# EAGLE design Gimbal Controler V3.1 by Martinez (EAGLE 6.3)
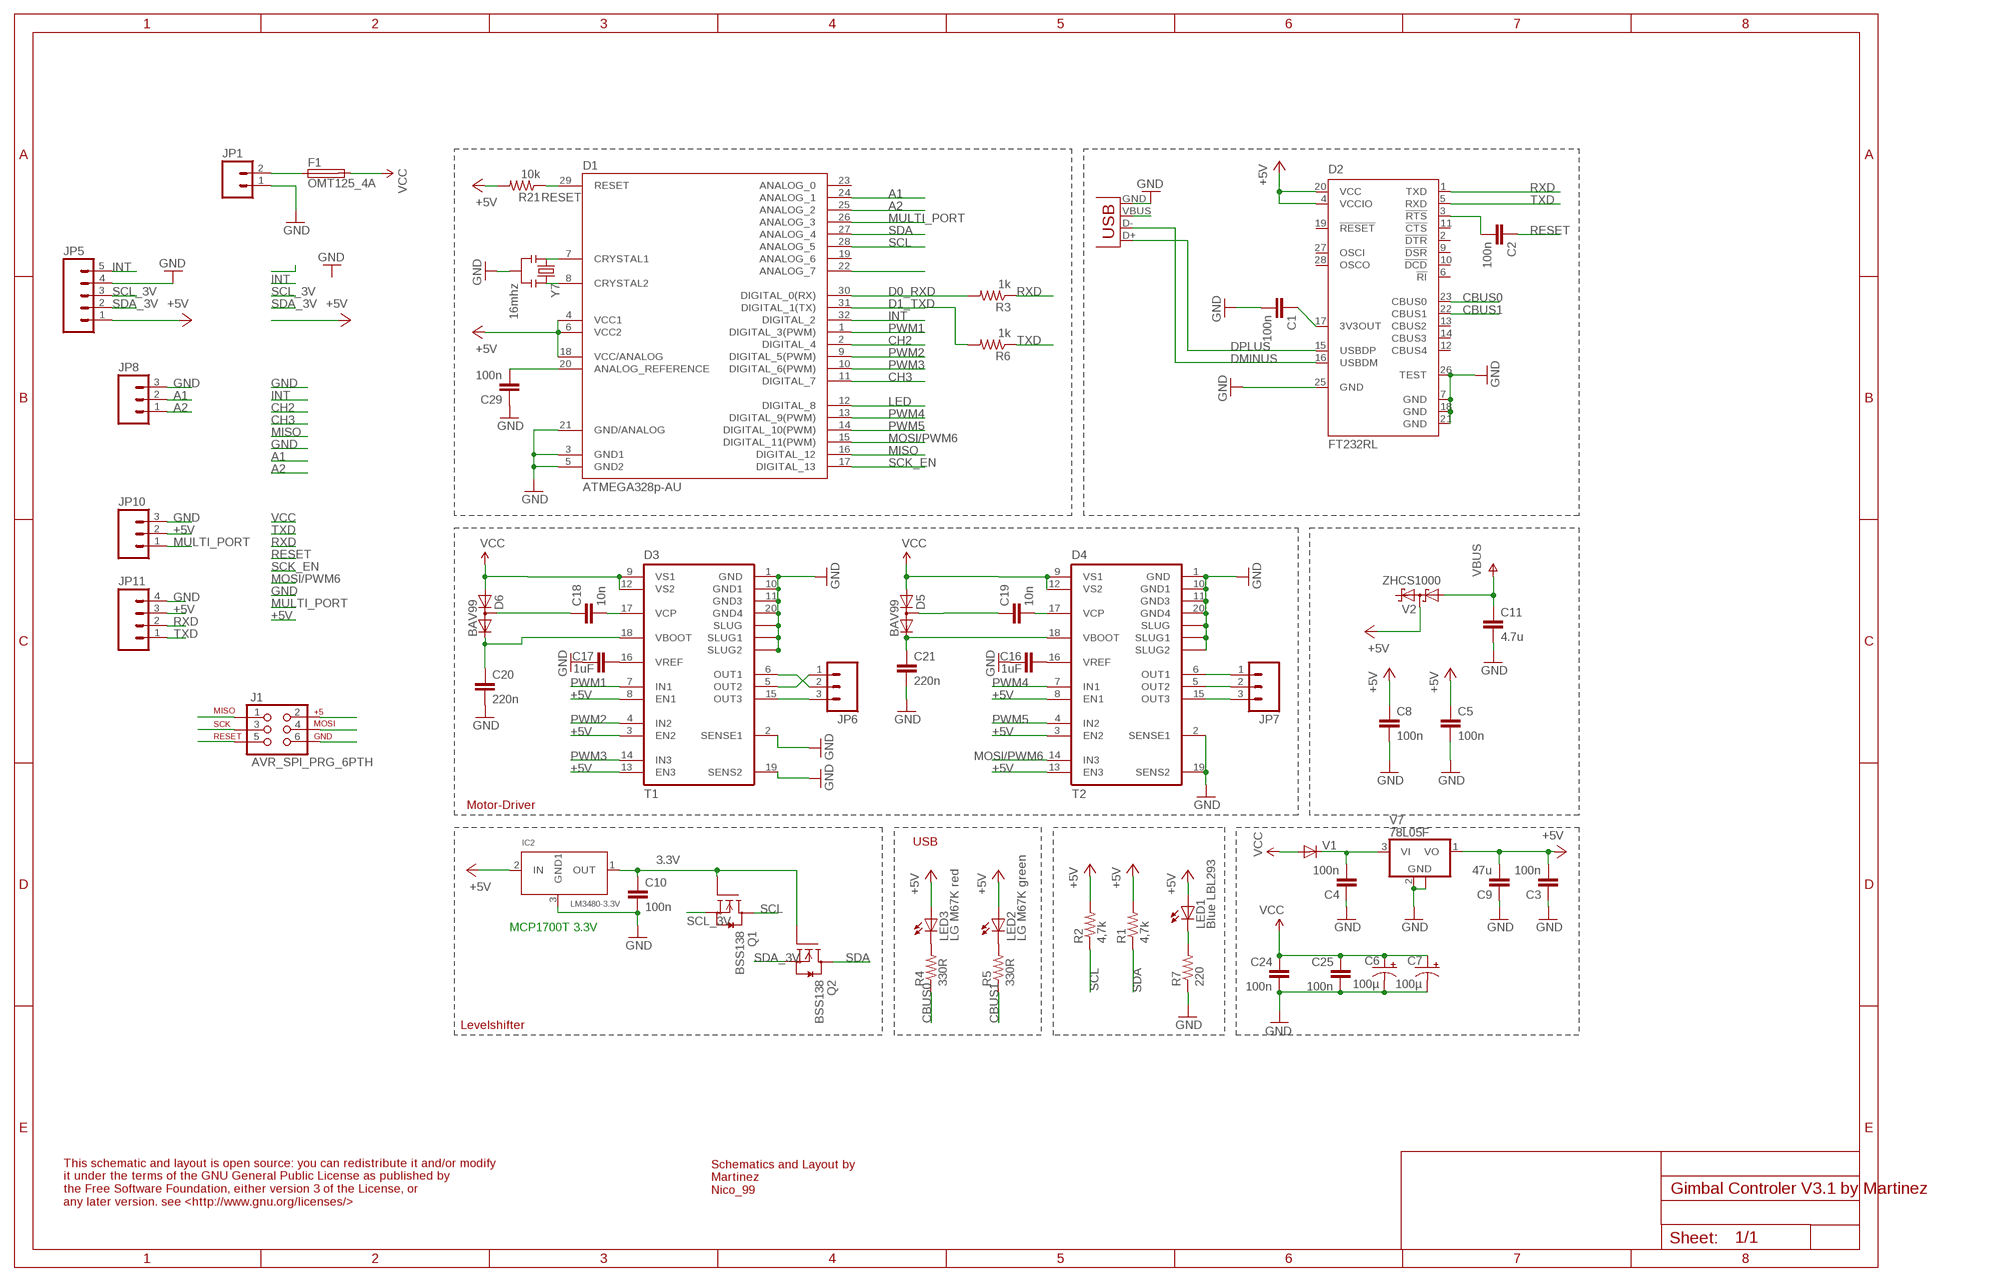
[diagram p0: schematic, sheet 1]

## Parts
C1  100n  CAP0805  [0805]
C2  100n  CAP0805  [0805]
C3  100n  CAP0805  [0805]
C4  100n  CAP0805  [0805]
C5  100n  CAP0805  [0805]
C6  100µ  CAP_POLD  [PANASONIC_D]
C7  100µ  CAP_POLD  [PANASONIC_D]
C8  100n  CAP0805  [0805]
C9  47u  C-EUC1210  [C1210]
C10  100n  CAP0805  [0805]
C11  4.7u  CAP0805  [0805]
C16  1uF  CAP0805  [0805]
C17  1uF  CAP0805  [0805]
C18  10n  CAP0805  [0805]
C19  10n  CAP0805  [0805]
C20  220n  CAP0805  [0805]
C21  220n  CAP0805  [0805]
C24  100n  CAP0805  [0805]
C25  100n  CAP0805  [0805]
C29  100n  CAP0805  [0805]
D1  ATMEGA328p-AU  ATMEGA168-AU  [TQFP32-08]
D2  FT232RL  [SSOP28]
D3  T1  L6234  [SO20POWER2]
D4  T2  L6234  [SO20POWER2]
D5  BAV99  BAV199  [SOT23]
D6  BAV99  BAV199  [SOT23]
F1  OMT125_4A  OMT125_11MM  [OMT125_11MM]
IC2  LM3480-3.3V  VREG_MULTI2  [SOT23]
J1  AVR_SPI_PRG_6PTH  [2X3]
JP1  M02PTH  [1X02]
JP5  M05PTH  [1X05]
JP6  M03PTH  [1X03]
JP7  M03PTH  [1X03]
JP8  M031X03_NO_SILK  [1X03_NO_SILK]
JP10  M031X03_NO_SILK  [1X03_NO_SILK]
JP11  M041X04_NO_SILK  [1X04_NO_SILK]
LED1  Blue LBL293  LEDCHIP-LED0603  [CHIP-LED0603]
LED2  LG M67K green  LEDCHIP-LED0805  [CHIP-LED0805]
LED3  LG M67K red  LEDCHIP-LED0805  [CHIP-LED0805]
Q1  BSS138  [SOT23]
Q2  BSS138  [SOT23]
R1  4,7k  RESISTOR0805-RES  [0805]
R2  4,7k  RESISTOR0805-RES  [0805]
R3  1k  RESISTOR0805-RES  [0805]
R4  330R  RESISTOR0805-RES  [0805]
R5  330R  RESISTOR0805-RES  [0805]
R6  1k  RESISTOR0805-RES  [0805]
R7  220  RESISTOR0805-RES  [0805]
R21  10k  RESISTOR0805-RES  [0805]
V1  DIODE-DO214AC  [DO214AC]
V2  ZHCS1000  BAS40-04  [SOT23]
V7  78L05F  [SOT89]
X2  USBOLD  [USB-MINIB-OLD]
Y7  16mhz  RESONATORSMD  [RESONATOR-SMD]

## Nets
3.3V: C10.1 IC2.1(OUT) Q1.1(G) Q2.1(G)
+5V: C3.2 C5.1 C8.1 C9.2 D1.4(VCC1) D1.6(VCC2) D1.18(VCC/ANALOG) D2.4(VCCIO) D2.20(VCC) D3.3(EN2) D3.8(EN1) D3.13(EN3) D4.3(EN2) D4.8(EN1) D4.13(EN3) IC2.2(IN) J1.2 JP5.1 JP10.2 JP11.3 LED1.A LED2.A LED3.A R1.2 R2.2 R21.2 V2.3(C1A2) V7.1(VO)
A1: D1.24(ANALOG_1) JP8.2
A2: D1.25(ANALOG_2) JP8.1
A7: D1.22(ANALOG_7)
CBUS0: D2.23(CBUS0) R4.1
CBUS1: D2.22(CBUS1) R5.1
CH2: D1.2(DIGITAL_4)
CH3: D1.11(DIGITAL_7)
D0_RXD: D1.30(DIGITAL_0(RX)) R3.2
D1_TXD: D1.31(DIGITAL_1(TX)) R6.2
DMINUS: D2.16(USBDM) X2.D-
DPLUS: D2.15(USBDP) X2.D+
GND: C1.2 C3.1 C4.1 C5.2 C6.- C7.- C8.2 C9.1 C10.2 C11.2 C16.1 C17.1 C20.2 C21.2 C24.2 C25.2 C29.1 D1.3(GND1) D1.5(GND2) D1.21(GND/ANALOG) D2.7(GND) D2.18(GND) D2.21(GND) D2.25(GND) D2.26(TEST) D3.1(GND) D3.2(SENSE1) D3.10(GND1) D3.11(GND3) D3.19(SENS2) D3.20(GND4) D3.SLUG1(SLUG2) D3.SLUG2(SLUG) D3.SLUG(SLUG1) D4.1(GND) D4.2(SENSE1) D4.10(GND1) D4.11(GND3) D4.19(SENS2) D4.20(GND4) D4.SLUG1(SLUG2) D4.SLUG2(SLUG) D4.SLUG(SLUG1) IC2.3(GND1) J1.6 JP1.1 JP5.4 JP8.3 JP10.3 JP11.4 R7.1 V7.2(GND) V7.2@1(GND) X2.GND Y7.2
INT: D1.32(DIGITAL_2) JP5.5
LED: D1.12(DIGITAL_8)
MISO: D1.16(DIGITAL_12) J1.1
MOSI/PWM6: D1.15(DIGITAL_11(PWM)) D4.14(IN3) J1.4
MULTI_PORT: D1.26(ANALOG_3) JP10.1
N$1: LED3.C R4.2
N$2: LED2.C R5.2
N$3: F1.P$1 JP1.2
N$4: LED1.C R7.2
N$7: C16.2 D4.16(VREF)
N$8: C17.2 D3.16(VREF)
N$17: C18.2 D3.17(VCP)
N$18: C19.2 D4.17(VCP)
N$19: C19.1 D5.3(AC)
N$20: C21.1 D4.18(VBOOT) D5.2(C)
N$21: D3.15(OUT3) JP6.3
N$22: C1.1 D2.17(3V3OUT)
N$23: D4.6(OUT1) JP7.1
N$24: D4.5(OUT2) JP7.2
N$25: D4.15(OUT3) JP7.3
N$26: C2.2 D2.3(!RTS)
N$27: D3.5(OUT2) JP6.1
N$28: D3.6(OUT1) JP6.2
N$38: D1.8(CRYSTAL2) Y7.3
N$39: D1.7(CRYSTAL1) Y7.1
N$40: C29.2 D1.20(ANALOG_REFERENCE)
PWM1: D1.1(DIGITAL_3(PWM)) D3.7(IN1)
PWM2: D1.9(DIGITAL_5(PWM)) D3.4(IN2)
PWM3: D1.10(DIGITAL_6(PWM)) D3.14(IN3)
PWM4: D1.13(DIGITAL_9(PWM)) D4.7(IN1)
PWM5: D1.14(DIGITAL_10(PWM)) D4.4(IN2)
RESET: C2.1 D1.29(RESET) J1.5 R21.1
RXD: D2.1(TXD) JP11.2 R3.1
SCK_EN: D1.17(DIGITAL_13) J1.3
SCL: D1.28(ANALOG_5) Q1.3(D) R2.1
SCL_3V: JP5.3 Q1.2(S)
SDA: D1.27(ANALOG_4) Q2.3(D) R1.1
SDA_3V: JP5.2 Q2.2(S)
TXD: D2.5(RXD) JP11.1 R6.1
VBOOT1: C20.1 D3.18(VBOOT) D6.2(C)
VBUS: C11.1 V2.1(A1) X2.VBUS
VCC: C6.+ C7.+ C24.1 C25.1 D3.9(VS1) D3.12(VS2) D4.9(VS1) D4.12(VS2) D5.1(A) D6.1(A) F1.P$2 V1.A
VCC_VI: C4.2 V1.C V7.3(VI)
VCP1: C18.1 D6.3(AC)
Unconnected: D1.19(ANALOG_6) D1.23(ANALOG_0) D2.2(!DTR) D2.6(!RI) D2.9(!DSR) D2.10(!DCD) D2.11(!CTS) D2.12(CBUS4) D2.13(CBUS2) D2.14(CBUS3) D2.19(!RESET) D2.27(OSCI) D2.28(OSCO) V2.2(C2)

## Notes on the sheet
- FTDI
- Motor-Driver
- USB
- MCP1700T 3.3V
- Levelshifter
- Schematics and Layout by
  Martinez
  Nico_99
- This schematic and layout is open source: you can redistribute it and/or modify
  it under the terms of the GNU General Public License as published by
  the Free Software Foundation, either version 3 of the License, or
  any later version. see <http://www.gnu.org/licenses/>

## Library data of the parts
C1-C5 C8 C10 C11 C16-C21 C24 C25 C29 = SparkFun:CAP: Capacitor
C6 C7 = SparkFun:CAP_POL: Capacitor Polarized
C9 = rcl:C-EU: CAPACITOR, European symbol
D1 = Arduino-AVR:ATMEGA168
D2 = ftdichip:FT232R: Source: http://www.ftdichip.com/Documents/DataSheets/DS_FT232R_v104.pdf; MPN: FT232RL; OC_FARNELL: 1146032; OC_NEWARK: 91K9918
D3 D4 = L6234:L6234
D5 D6 = diode:BAV199: DIODE low-leakage double diode
F1 = fuse:OMT125_11MM
IC2 = m-pad-2.1_my:VREG_MULTI2: standard package voltage regulator (LM3480, etc)
J1 = SparkFun:AVR_SPI_PRG_6: AVR ISP 6 Pin This is the reduced ISP connector for AVR programming. Common on Arduino. This footprint will take up less PCB space and can be used with a 10-pin to 6-pin adapter such as SKU: BOB-08508
JP1 = SparkFun:M02: Header 2
JP5 = SparkFun:M05: Header 5 Standard 5-pin 0.1" header. Use with straight break away headers (SKU : PRT-00116), right angle break away headers (PRT-00553), swiss pins (PRT-00743), machine pins (PRT-00117), and female headers (PRT-00115). Molex polarized connector foot print use with SKU : PRT-08230 with associated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
JP6-JP8 JP10 = SparkFun:M03: Header 3 Standard 3-pin 0.1" header. Use with straight break away headers (SKU : PRT-00116), right angle break away headers (PRT-00553), swiss pins (PRT-00743), machine pins (PRT-00117), and female headers (PRT-00115). Molex polarized connector foot print use with SKU : PRT-08232 with associated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
JP11 = SparkFun:M04: Header 4 Standard 4-pin 0.1" header. Use with straight break away headers (SKU : PRT-00116), right angle break away headers (PRT-00553), swiss pins (PRT-00743), machine pins (PRT-00117), and female headers (PRT-00115). Molex polarized connector foot print use with SKU : PRT-08231 with associated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
LED1-LED3 = led:LED: LED
Q1 Q2 = m-pad-2.1_my:BSS138: Fairchild Semiconductors BSS138 N-Channel Logic Level Enhancement Mode Field Effect Transistor General Description: These N-Channel enhancement mode field effect transistors are produced using Fairchild's proprietary, high cell density, DMOS technology. These products have been designed to minimize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
R1-R7 R21 = SparkFun:RESISTOR: Resistor
V1 = diode:DIODE-: DIODE
V2 = diode:BAS40-04: Silicon Schottky Diodes General-purpose diode for high-speed switching
V7 = linear:78L*: POSITOIV-VOLTAGE REGULATORS Output up to 100 mA Source: http://focus.ti.com/lit/ds/symlink/ua78l05.pdf
X2 = SparkFun:USB: USB Connectors USB-B-PTH is fully proven SKU : PRT-00139 USB-miniB is fully proven SKU : PRT-00587 USB-A-PCB is untested. USB-A-H is throughly reviewed, but untested. Spark Fun Electronics SKU : PRT-00437 USB-B-SMT is throughly reviewed, but untested. Needs silkscreen touching up. USB-A-S has not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
Y7 = SparkFun:RESONATOR: Resonator Small SMD resonator. This is the itty bitty 10/20MHz resonators with built in caps. CSTCE10M0G55 and CSTCE20M0V53. Footprint has been reviewed closely but hasn't been tested yet.

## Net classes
0 default: width 0.152 mm, clearance 0.152 mm

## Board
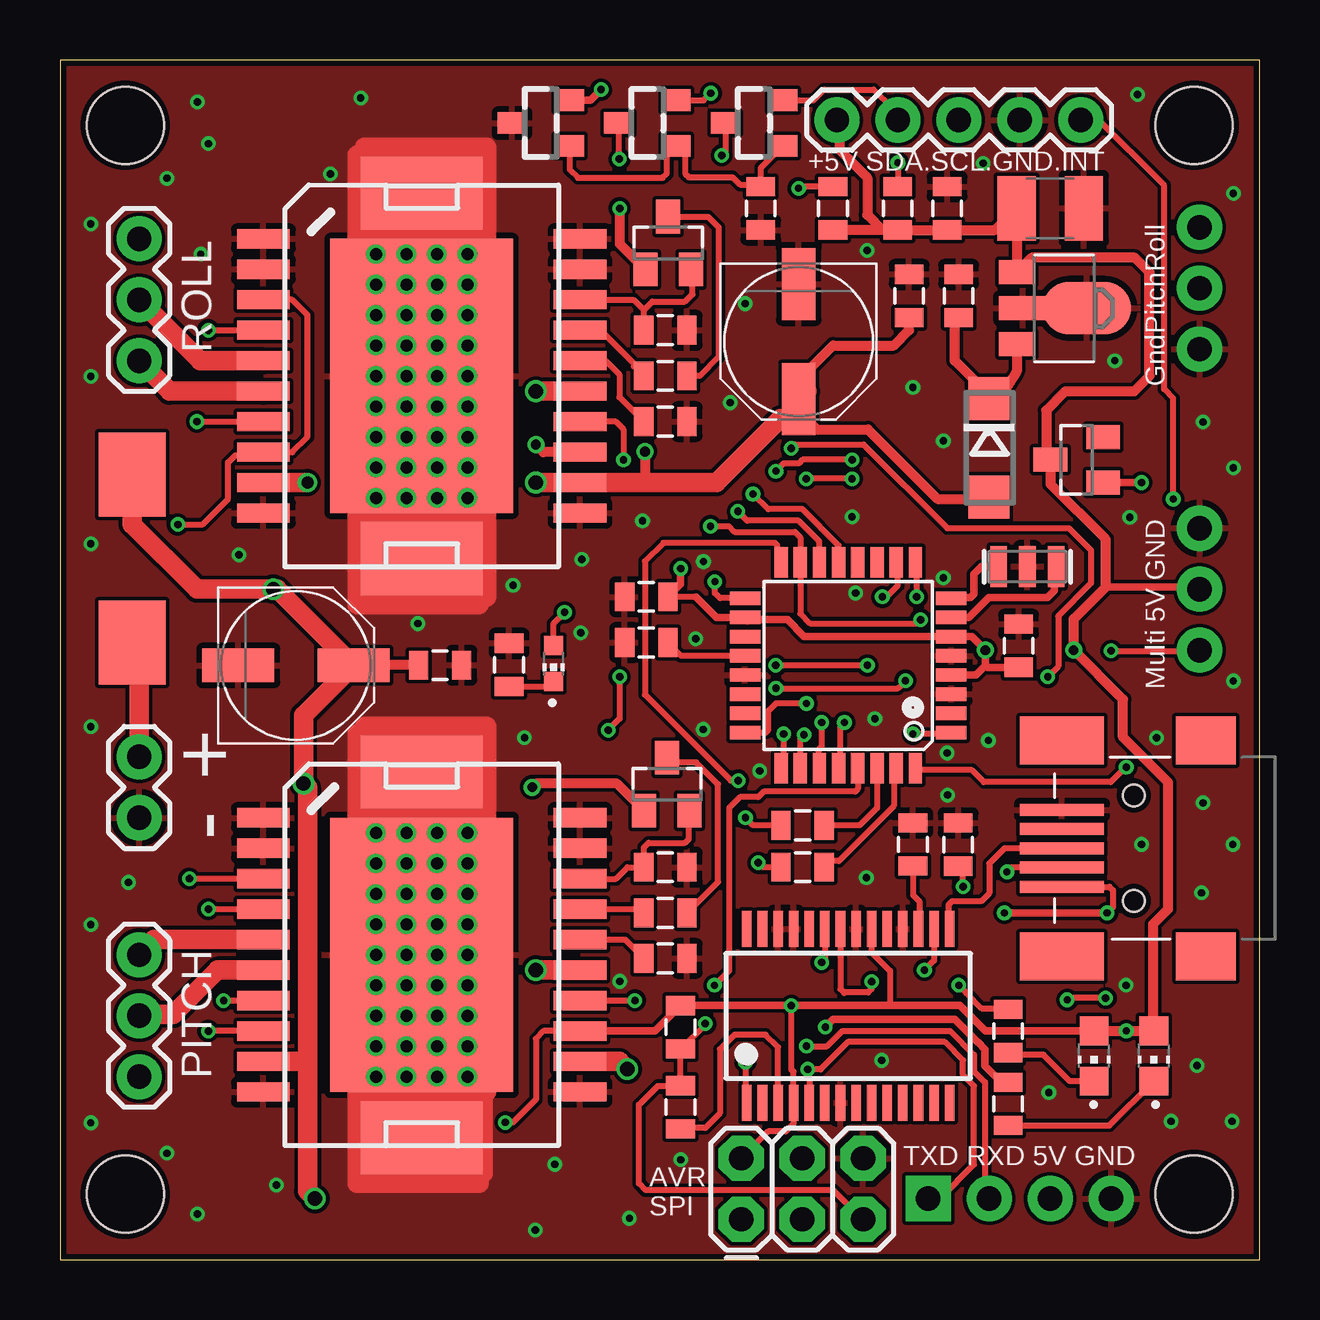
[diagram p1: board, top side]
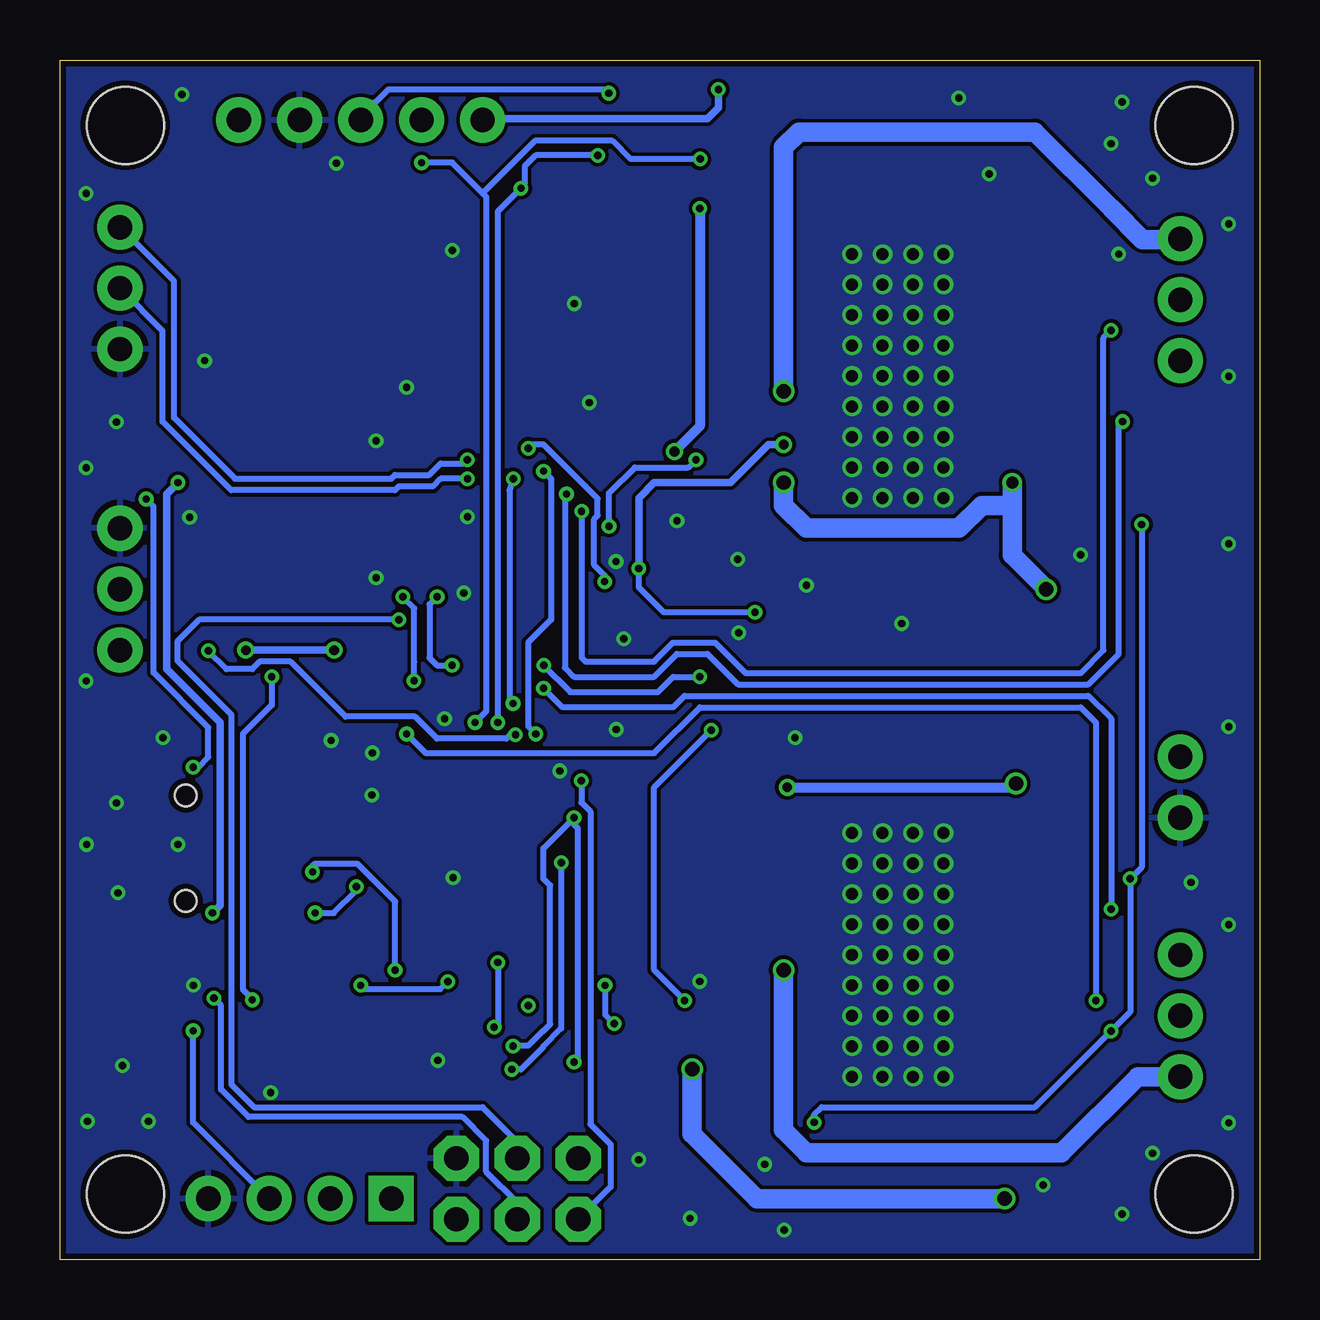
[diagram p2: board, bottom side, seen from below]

Size 50 x 50 mm. Coordinates in mm from the lower left corner, seen from the top.
Outline: 50,0 50,50 0,50 0,0 50,0
Copper layers (1*16): Top 0.035mm / dielectric 1.5mm / Bottom 0.035mm
Design rules "ITEADstudio_DRC *": minimum track width 6mil, minimum drill 12mil, track to track 6mil, track to pad 6mil, pad to pad 6mil, via to via 6mil, smd to smd 0mil, copper to edge 10mil, drill to drill 10mil, minimum pad ring 10mil, minimum via ring 6mil, stop-mask expansion 2mil, vias tented up to drill 100mil, thermal gap 10mil
Holes 3.2 mm at 47.27,2.73 2.73,2.73 2.73,47.27 47.27,47.27

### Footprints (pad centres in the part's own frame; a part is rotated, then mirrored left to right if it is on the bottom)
0805 = smd 0.8 x 1.2: 1 -0.9,0; 2 0.9,0
PANASONIC_D = smd 3 x 1.4: + 2.4,0; - -2.4,0
C1210 = smd 1.6 x 2.7: 1 -1.4,0; 2 1.4,0
TQFP32-08 = smd 1.27 x 0.559: 1 -4.293,2.8; 2 -4.293,2; 3 -4.293,1.2; 4 -4.293,0.4; 5 -4.293,-0.4; 6 -4.293,-1.2; 7 -4.293,-2; 8 -4.293,-2.8; 17 4.293,-2.8; 18 4.293,-2; 19 4.293,-1.2; 20 4.293,-0.4; 21 4.293,0.4; 22 4.293,1.2; 23 4.293,2; 24 4.293,2.8 | smd 0.559 x 1.27: 9 -2.8,-4.293; 10 -2,-4.293; 11 -1.2,-4.293; 12 -0.4,-4.293; 13 0.4,-4.293; 14 1.2,-4.293; 15 2,-4.293; 16 2.8,-4.293; 25 2.8,4.293; 26 2,4.293; 27 1.2,4.293; 28 0.4,4.293; 29 -0.4,4.293; 30 -1.2,4.293; 31 -2,4.293; 32 -2.8,4.293
SSOP28 = smd 0.4 x 1.5: 1 -4.225,-3.625; 2 -3.575,-3.625; 3 -2.925,-3.625; 4 -2.275,-3.625; 5 -1.625,-3.625; 6 -0.975,-3.625; 7 -0.325,-3.625; 8 0.325,-3.625; 9 0.975,-3.625; 10 1.625,-3.625; 11 2.275,-3.625; 12 2.925,-3.625; 13 3.575,-3.625; 14 4.225,-3.625; 15 4.225,3.625; 16 3.575,3.625; 17 2.925,3.625; 18 2.275,3.625; 19 1.625,3.625; 20 0.975,3.625; 21 0.325,3.625; 22 -0.325,3.625; 23 -0.975,3.625; 24 -1.625,3.625; 25 -2.275,3.625; 26 -2.925,3.625; 27 -3.575,3.625; 28 -4.225,3.625
SO20POWER2 = smd 0.8 x 2.2: 1 -5.715,-6.6; 2 -4.445,-6.6; 3 -3.175,-6.6; 4 -1.905,-6.6; 5 -0.635,-6.6; 6 0.635,-6.6; 7 1.905,-6.6; 8 3.175,-6.6; 9 4.445,-6.6; 10 5.715,-6.6; 11 5.715,6.6; 12 4.445,6.6; 13 3.175,6.6; 14 1.905,6.6; 15 0.635,6.6; 16 -0.635,6.6; 17 -1.905,6.6; 18 -3.175,6.6; 19 -4.445,6.6; 20 -5.715,6.6 | smd 3.048 x 5.08: SLUG -7.62,0; SLUG2 7.62,0 | smd 11.43 x 7.62: SLUG1 0,0
SOT23 = smd 1 x 1.4: 1 -0.95,-1.1; 2 0.95,-1.1; 3 0,1.1
OMT125_11MM = smd 3.5 x 2.8: P$1 -3.5,0; P$2 3.5,0
SOT23' = smd 0.9 x 1.2: 1 -0.95,-1.2; 2 0.95,-1.2; 3 0,1.2
2X3 = drill 1.016 pad 1.88 octagon: 1 0,0; 2 0,2.54; 3 2.54,0; 4 2.54,2.54; 5 5.08,0; 6 5.08,2.54
1X02 = drill 1.016 pad 1.88: 1 0,0; 2 2.54,0
1X05 = drill 1.016 pad 1.88: 1 0,0; 2 2.54,0; 3 5.08,0; 4 7.62,0; 5 10.16,0
1X03 = drill 1.016 pad 1.88: 1 0,0; 2 2.54,0; 3 5.08,0
1X03_NO_SILK = drill 1.016 pad 1.88: 1 0,0; 2 2.54,0; 3 5.08,0
1X04_NO_SILK = drill 1.016 pad 1.88 square: 1 0,0 | drill 1.016 pad 1.88: 2 2.54,0; 3 5.08,0; 4 7.62,0
CHIP-LED0603 = smd 0.8 x 0.8: A 0,-0.75; C 0,0.75
CHIP-LED0805 = smd 1.2 x 1.2: A 0,-1.05; C 0,1.05
DO214AC = smd 1.8 x 1.7: A 2.05,0; C -2.05,0
SOT89 = smd 1 x 1.5: 1 -1.499,-1.981; 3 1.499,-1.981 | smd 1 x 2: 2 0,-1.727 | smd 2.2 x 3.7: 2@1 0,0.94
USB-MINIB-OLD = smd 2.5 x 2: 1 -3,-4.5; 2 -3,4.5 | smd 3.5 x 2: 3 3,-4.5; 4 3,4.5 | smd 3.5 x 0.5: D+ 3,0; D- 3,0.8; GND 3,-1.6; ID 3,-0.8; VBUS 3.01,1.61 | hole 0.9: 0,2.2; 0,-2.2
RESONATOR-SMD = smd 0.7 x 1.7: 1 -1.2,0; 2 0,0; 3 1.2,0

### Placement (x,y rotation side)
C1  35.55,17.3 90 top
C2  25.87,6.35 270 top
C3  36.98,43.81 270 top
C4  37.46,40.16 270 top
C5  24.44,27.62 180 top
C6  9.84,24.77 0 top
C7  30.79,38.26 270 top
C8  39.96,25.58 90 top
C9  41.27,43.81 180 top
C10  29.21,43.81 270 top
C11  37.44,17.3 90 top
C16  25.23,34.92 180 top
C17  25.23,12.55 180 top
C18  25.23,14.45 180 top
C19  25.23,36.83 180 top
C20  25.23,16.35 0 top
C21  25.23,38.73 0 top
C24  35.4,40.16 90 top
C25  15.84,24.77 0 top
C29  24.44,25.72 0 top
D1  32.85,24.77 180 top
D2  32.85,10.16 0 top
D3  15.07,12.7 270 top
D4  15.07,36.83 270 top
D5  25.35,42.37 0 top
D6  25.3,19.81 0 top
F1  3.01,29.21 90 top
IC2  LM3480-3.3V  [SOT23']  20.04,47.37 90 top
J1  28.4,1.68 0 top
JP1  3.3,18.41 90 top
JP5  32.38,47.5 0 top
JP6  3.3,12.7 270 top
JP7  3.3,37.47 90 top
JP8  47.5,43.03 270 top
JP10  47.5,25.4 90 top
JP11  36.2,2.54 0 top
LED1  20.57,24.84 180 top
LED2  43.1,8.48 180 top
LED3  45.59,8.48 180 top
Q1  BSS138  [SOT23']  24.49,47.37 90 top
Q2  BSS138  [SOT23']  28.93,47.37 90 top
R1  32.22,43.81 270 top
R2  34.92,43.81 270 top
R3  30.95,18.1 0 top
R4  39.52,6.49 270 top
R5  39.52,9.53 270 top
R6  30.95,16.35 0 top
R7  18.72,24.79 270 top
R21  25.87,9.68 90 top
V1  38.72,33.83 270 top
V2  42.38,33.34 90 top
V7  41.87,39.65 270 top
X2  44.76,17.14 180 top
Y7  40.32,28.88 180 top

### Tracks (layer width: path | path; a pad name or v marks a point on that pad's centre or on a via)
3.3V
  Top 0.254: IC2.1 21.24,45.43 21.59,45.09 25.12,45.09 25.3,45.26 25.3,46.03 Q1.1 25.82,46.42 26.06,46.18 26.06,45.26 26.21,45.11 28.04,45.11 28.35,44.81 29.12,44.81 C10.1 29.21,45.5 Q2.1
+5V  (via drill 0.3, 0.41)
  Top 0.254: 28.63,26.83 D1.18 | D4.3 9.68,40.01 10.31,39.37 10.31,34.29 9.68,33.66 D4.8 8.35,33.53 7.32,33.53 7.01,33.22 7.01,31.7 5.95,30.64 v4.92,30.64 | D3.13 20.16,9.53 19.84,9.21 19.84,6.67 18.89,5.71 v18.57,5.71 | D3.8 v6.18,9.53 | D3.3 v5.39,15.88 | 26.5,27.62 C5.1 25.4,27.68 | LED1.A 20.57,26.52 v21.03,26.98 | D2.20 33.83,12.8 34.59,12.04 34.59,10.58 | J1.2 29.52,5.33 30.25,5.33 30.58,5.66 D2.4 30.58,7.83 30.48,7.92 v30.48,10.58
  Top 0.305: D1.4 38.17,24.36 38.57,24.77 | 38.57,24.77 v38.57,25.4 38.01,25.96 D1.6 31.02,25.96 30.32,26.67 28.66,26.67 | D1.18 27.36,26.77 26.5,27.62 | D3.13 24.81,9.53 R21.2 v30.48,10.58 34.59,10.58 37.51,10.58 38.57,9.53 43.02,9.53 | IC2.2 22.11,48.32 v22.55,48.77 | C8.1 38.65,24.68 38.57,24.77 | v25.87,28.8 25.87,28.15 C5.1 | 43.59,28.04 47.4,28.04 JP10.2
  Top 0.406: D4.13 20.16,33.66 v19.84,33.97 | 28.66,26.67 D1.18 | V2.3 41.11,33.51 41.11,35.4 41.91,36.2 44.78,36.2 45.41,36.83 45.41,41.15 44.81,41.76 40.49,41.76 V7.1 39.88,41.46 C9.2 38.98,42.91 C3.2 R2.2 34.29,42.91 | 41.11,33.17 V2.3 | 34.29,42.91 R1.2 | 34.29,42.91 33.66,43.55 33.66,45.09 32.5,46.24 32.5,47.38 JP5.1 | V2.3 41.3,33.32 41.3,32.31 43.59,30.02 43.59,28.04 42.25,26.71 v42.25,25.4 44.3,23.35 44.3,21.77 46.19,19.89 46.19,14.61 45.55,13.97 45.55,9.57 LED3.A v44.45,9.53 LED2.A 43.02,9.53
  Bottom 0.254: v4.92,30.64 4.92,16.35 v5.39,15.88 5.39,10.32 v6.18,9.53 9.36,6.35 18.25,6.35 18.57,6.03 v18.57,5.71 | 38.73,25.24 v38.57,25.4 | v21.03,26.98 24.83,26.98 25.87,28.02 v25.87,28.8 | JP11.3 44.45,5.71 v44.45,9.53
  Bottom 0.305: v38.57,25.4 v42.25,25.4 | v19.84,33.97 20.47,33.97 22.06,32.38 25.23,32.38 25.87,31.75 v25.87,28.8 | v22.55,48.77 22.55,48.01 23.01,47.55 32.34,47.55 JP5.1
A1  (via drill 0.3)
  Top 0.254: v33.01,32.54 v31.11,32.54 | 28.66,22.07 D1.24 29.43,21.96 29.53,22.07 29.53,22.86 29.84,23.18 v31.11,23.18
  Bottom 0.254: v31.11,32.54 31.27,32.07 31.27,23.33 v31.11,23.18 | v33.01,32.54 34.13,32.54 34.45,32.23 35.88,32.23 36.04,32.07 42.86,32.07 45.72,34.92 45.72,38.71 JP8.2
A2  (via drill 0.3)
  Top 0.254: v33.02,33.34 30.96,33.34 30.8,33.18 30.16,33.18 v29.84,32.86 | v30.16,21.91 30.16,20.58 D1.25
  Bottom 0.254: v33.02,33.34 33.18,33.18 34.13,33.18 34.61,32.7 36.04,32.7 36.2,32.54 42.7,32.54 45.24,35.08 45.24,40.77 JP8.1 | v29.84,32.86 29.53,32.54 29.53,26.67 30.48,25.72 30.48,22.23 v30.16,21.91
CBUS0  (via drill 0.3)
  Top 0.254: D2.23 31.88,12.52 v31.74,12.38
  Top 0.305: v31.9,9.68 32.22,10 37.3,10 38.25,9.05 38.27,9.05 38.56,8.76 38.56,8.08 39.01,7.62 39.29,7.62 R4.1 39.45,7.32
  Bottom 0.254: v31.74,12.38 31.74,9.84 v31.9,9.68
CBUS1  (via drill 0.3)
  Top 0.254: D2.22 32.53,11.28 32.7,11.11 32.71,11.12 33.68,11.12 33.83,11.28 v33.83,11.58 | R5.1 39.47,10.48 38.41,10.48 37.78,11.11 37.78,11.12 v37.47,11.43
  Bottom 0.254: v37.47,11.43 37.47,11.4 37.34,11.28 34.14,11.28 v33.83,11.58
D0_RXD
  Top 0.254: D1.30 34.05,18.82 33.33,18.1 R3.2
D1_TXD
  Top 0.254: D1.31 34.85,20.41 34.76,20.32 34.76,18.91 32.46,16.61 32.11,16.61 R6.2
DMINUS  (via drill 0.3)
  Top 0.254: D2.16 36.43,12.46 v36.03,12.06 | X2.D- 39.66,16.34 v39.47,16.15
  Bottom 0.254: v36.03,12.06 36.03,14.92 37.62,16.51 39.37,16.51 39.47,16.41 v39.47,16.15
DPLUS
  Top 0.254: D2.15 37.03,13.83 37.03,14.78 37.19,14.94 38.41,14.94 38.73,15.27 38.73,16.51 39.37,17.14 X2.D+
GND  (via drill 0.3, 0.5)
  Top 0.508: 17.78,6.99 17.78,3.49
  Top 0.813: 12.7,46.35 17.78,46.35 17.78,42.55 12.38,42.55 12.38,46.04 | 17.46,27.3 12.38,27.3 12.38,31.11 17.78,31.11 17.78,27.62 | 12.7,22.23 17.78,22.23 17.78,18.41 12.38,18.41 12.38,21.91 | 17.46,3.17 12.38,3.17 12.38,6.99 17.78,6.99
  other vias: 4.46,4.43 44.92,48.56 13.17,12.7 13.17,11.43 13.17,10.16 13.17,8.89 13.17,7.62 14.44,7.62 14.44,8.89 14.44,10.16 14.44,11.43 14.44,12.7 15.71,10.16 15.71,8.89 15.71,7.62 16.98,7.62 16.98,8.89 16.98,10.16 15.71,11.43 15.71,12.7 16.98,12.7 16.98,11.43 15.71,13.97 15.71,15.24 15.71,16.51 15.71,17.78 13.17,13.97 13.17,15.24 13.17,16.51 13.17,17.78 14.44,13.97 14.44,15.24 14.44,16.51 14.44,17.78 16.98,13.97 16.98,15.24 16.98,16.51 16.98,17.78 13.17,35.56 13.17,34.29 13.17,33.02 13.17,31.75 14.44,31.75 14.44,33.02 14.44,34.29 14.44,35.56 15.71,34.29 15.71,33.02 15.71,31.75 16.98,31.75 16.98,33.02 16.98,34.29 15.71,35.56 16.98,35.56 13.17,41.91 13.17,40.64 13.17,39.37 13.17,38.1 14.44,38.1 14.44,39.37 14.44,40.64 14.44,41.91 15.71,40.64 15.71,39.37 15.71,38.1 16.98,38.1 16.98,39.37 16.98,40.64 15.71,41.91 16.98,41.91 13.17,36.83 14.44,36.83 15.71,36.83 16.98,36.83 28.57,39.85 36.82,34.13 33.97,22.54 35.55,36.35 26.5,25.88 23.34,11.6 14.92,26.51 33.01,30.96 36.82,28.42 27.93,35.72 33.65,42.07 33.17,27.78 37,19.36 45.08,17.3 45.71,21.75 21.76,29.18 24.28,30.8 2.85,15.72 5.87,41.91 6.18,46.51 36.98,21.11 44.44,11.43 43.97,37.47 41.22,6.96 12.54,48.42 11.27,45.24 7.46,29.37 18.89,28.1 19.36,21.75 20.63,3.97 9.02,3.11 19.82,1.23 47.39,8.08 44.6,30.94 38.48,45.69 26.81,22.09 48.89,17.3 21.7,26.13 29.17,20.36 38.7,21.63 33.62,15.92 47.59,15.28 34.25,8.3 25.87,4.16 23.74,1.72 26.82,29.1 5.73,1.89 1.28,5.7 1.28,13.96 1.28,22.21 1.28,29.83 1.28,36.81 1.28,43.16 5.73,48.24 4.46,45.07 48.91,44.44 47.64,34.91 48.91,33.01 48.91,24.11 47.64,19.04 48.86,5.76 46.32,5.76
  pour Top: 0.25,0.25 0.25,49.75 49.75,49.75 49.75,0.25
  pour Bottom: 0.25,0.25 0.25,49.75 49.75,49.75 49.75,0.25
INT  (via drill 0.3)
  Top 0.152: D1.32 35.56,20.32 35.6,20.3
  Top 0.254: v44.45,20.52 44.22,20.32 43.8,19.9 38.5,19.9 38,20.4 35.7,20.4 | v46.41,31.7 46.41,35.89 46.02,36.27 46.02,44.78 43.18,47.62 42.67,47.62 JP5.5
  Top 0.305: 35.7,20.4 35.6,20.3
  Bottom 0.254: v44.45,20.52 44.25,20.52 43.81,20.95 43.81,22.17 46.1,24.46 46.1,31.39 v46.41,31.7
MISO  (via drill 0.3)
  Top 0.254: v28.27,19.96 27.96,19.96 24.38,23.55 24.38,29.11 25.15,29.87 29.79,29.87 29.9,29.76 29.9,29.3 30.05,29.3 D1.16
  Bottom 0.254: v28.27,19.96 28.27,19.05 27.89,18.67 27.89,5.64 27.05,4.8 27.05,3.02 J1.1
MOSI/PWM6  (via drill 0.3)
  Top 0.254: D4.14 23.17,34.92 23.49,34.61 v23.49,33.34 | v35.87,26.67 35.71,26.51 31.27,26.51 30.86,26.92 D1.15 30.86,29.62 30.86,29.63 30.86,30.1 30.63,30.33 28.12,30.33 27.88,30.57 v27.11,30.57
  Bottom 0.254: v35.87,26.67 44.2,26.67 45.11,25.76 45.11,24.97 42.86,22.71 42.86,7.3 41.91,6.35 32.38,6.35 31.11,5.08 31.11,4.39 J1.4 | v27.11,30.57 27.11,31.94 26.04,33.02 23.81,33.02 v23.49,33.34
MULTI_PORT  (via drill 0.3)
  Top 0.254: D1.26 30.86,21.71 v31.01,21.87 | v43.81,25.38 47.48,25.38 JP10.1
  Bottom 0.254: v31.01,21.87 31.24,21.87 31.39,21.72 34.29,21.72 35.2,22.63 38.1,22.63 40.39,24.92 41.68,24.92 41.99,24.61 43.05,24.61 v43.81,25.38
N$1
  Top 0.254: R4.2 43.75,5.59 LED3.C
N$2
  Top 0.254: LED2.C 42.1,7.43 41,8.53 39.61,8.53 R5.2
N$3
  Top 0.813: JP1.2 3.3,25.42 F1.P$1
N$4
  Top 0.254: R7.2 20.37,23.89 LED1.C
N$7
  Top 0.254: D4.16 22.73,37.47 23.32,36.88 23.32,35.94 C16.2
N$8
  Top 0.254: D3.16 23.55,13.34 C17.2
N$17
  Top 0.254: D3.17 24.18,14.61 C18.2
N$18
  Top 0.254: D4.17 22.53,38.73 23.93,37.34 23.93,37.24 C19.2
N$19
  Top 0.254: D5.3 27.02,43.47 27.46,43.03 27.46,37.62 26.67,36.83 C19.1
N$20
  Top 0.254: D4.18 23.91,40.01 24.34,39.58 | C21.1 24.34,39.58 | 24.34,39.58 24.69,39.93 26.06,39.93 26.36,40.23 26.36,41.2 D5.2
N$21  (via drill 0.6)
  Top 0.813: D3.15 v19.84,12.06
  Bottom 0.813: v19.84,12.06 19.84,5.4 18.89,4.45 8.26,4.45 5.08,7.62 JP6.3
N$22
  Top 0.254: C1.1 35.55,15.2 35.81,14.94 35.81,13.82 D2.17
N$23
  Top 0.813: D4.6 4.57,36.2 JP7.1
N$24
  Top 0.813: D4.5 5.84,37.47 JP7.2
N$25  (via drill 0.6)
  Top 0.813: D4.15 v19.84,36.2
  Bottom 0.813: v19.84,36.2 19.84,46.35 19.2,46.99 9.36,46.99 6.18,43.81 6.17,43.81 4.88,42.52 3.33,42.52 JP7.3
N$26
  Top 0.254: D2.3 29.93,8.86 29.41,9.37 28.12,9.37 27.51,8.76 27.51,6.1 26.9,5.49 25.91,5.49 C2.2
N$27
  Top 0.813: D3.5 3.94,13.34 JP6.1
N$28
  Top 0.813: D3.6 6.58,12.06 4.72,10.21 3.35,10.21 JP6.2
N$38
  Top 0.305: Y7.3 38.41,28.88 38.1,28.57 38.1,27.74 37.95,27.58 37.17,27.58 D1.8
N$39
  Top 0.305: D1.7 37.89,26.77 38.71,27.58 41.15,27.58 41.45,27.89 41.45,28.81 Y7.1
N$40
  Top 0.254: D1.20 25.89,25.16 C29.2
PWM1  (via drill 0.3)
  Top 0.254: 8.32,10.95 D3.7 v6.82,10.79 | D1.1 37.09,21.91 v35.55,21.91
  Bottom 0.254: v6.82,10.79 6.82,22.38 7.46,23.02 23.33,23.02 25.23,21.11 34.76,21.11 v35.55,21.91
PWM2  (via drill 0.3)
  Top 0.254: v6.18,14.61 D3.4 | v35.71,27.62 35.71,29 D1.9 | v29.84,23.81 34.92,23.81 v35.24,24.13
  Bottom 0.254: v6.18,14.61 6.18,22.54 7.14,23.5 23.96,23.5 24.44,23.02 29.05,23.02 v29.84,23.81 | v35.71,27.62 35.24,27.15 35.24,24.92 v35.24,24.13
PWM3  (via drill 0.3)
  Top 0.254: D3.14 v23.96,10.79 | 34.76,28.96 D1.10 34.92,28.99 34.92,28.1 34.44,27.62 v34.28,27.62 | v23.33,24.29 23.33,22.54 v22.85,22.07 | v33.66,24.77 v29.84,24.77
  Bottom 0.254: v23.96,10.79 25.23,12.06 25.23,19.68 v22.85,22.07 | v23.33,24.29 24.44,24.29 25.08,23.65 28.73,23.65 v29.84,24.77 | v34.28,27.62 34.6,27.3 34.6,25.08 34.29,24.77 v33.66,24.77
PWM4  (via drill 0.3)
  Top 0.254: D1.13 32.45,29.77 30.95,31.27 29.52,31.27 v28.89,31.91 | v5.71,34.92 D4.7
  Bottom 0.254: v5.71,34.92 5.87,34.77 5.87,25.24 7.14,23.97 21.74,23.97 23.01,25.24 24.28,25.24 25.23,24.29 28.57,24.29 28.96,24.68 28.96,31.85 v28.9,31.91 v28.89,31.91
PWM5  (via drill 0.3)
  Top 0.254: v6.18,38.73 D4.4 | D1.14 31.66,29.93 30.79,30.8 28.64,30.8 v28.26,31.18
  Bottom 0.254: v6.18,38.73 6.5,38.42 6.5,25.4 7.46,24.45 21.43,24.45 22.7,25.72 24.44,25.72 25.23,24.92 28.09,24.92 28.26,25.09 v28.26,31.18
RESET  (via drill 0.3)
  Top 0.254: J1.5 33.45,1.68 32.23,2.9 24.41,2.9 24.13,3.17 24.13,6.45 24.92,7.24 C2.1 R21.1 26.9,9.81 v26.9,9.83 | v27.28,11.43 27.89,12.04 27.89,18.82 28.35,19.28 29.11,19.28 29.34,19.51 33.15,19.51 33.26,19.61 D1.29
  Bottom 0.254: v27.28,11.43 27.28,10.21 v26.9,9.83
RXD  (via drill 0.3)
  Top 0.254: R3.1 28.89,18.1 v28.57,18.41 | v28.57,8.23 28.57,6.59 D2.1 | v31.11,8.89 31.98,8.89 32.61,9.53 37.11,9.53 38.1,8.53 38.1,7.85 38.56,7.39 38.56,2.72 JP11.2
  Bottom 0.254: v31.11,8.89 31.09,8.91 30.48,8.91 29.87,9.53 29.84,9.53 29.57,9.8 29.57,15.6 29.84,15.88 29.84,17.14 v28.57,18.41 28.57,18.14 28.42,17.98 28.42,8.38 v28.57,8.23
SCK_EN  (via drill 0.3)
  Top 0.254: D1.17 27.52,27.57 27.3,27.78 v27.3,28.26 | v30.48,33.81 30.64,33.97 33.49,33.97 36.98,30.48 42.06,30.48 42.98,29.57 42.98,28.19 41.6,26.82 41.6,24.72 v41.17,24.29 41.15,24.31 | v43.59,10.9 42.06,10.9 v41.99,10.82
  Bottom 0.254: v30.48,33.81 30.32,33.97 29.84,33.97 28.1,32.23 28.09,32.23 27.58,31.72 27.58,31.01 27.74,30.86 27.74,28.96 27.3,28.52 v27.3,28.26 | v41.17,24.29 41.17,23.11 42.38,21.91 42.38,11.27 41.99,10.87 v41.99,10.82 | J1.3 30.94,2.36 32.23,3.66 32.23,4.95 33.22,5.94 42.14,5.94 43.28,7.09 43.28,10.59 v43.59,10.9
SCL  (via drill 0.3)
  Top 0.254: D1.28 32.54,20.55 32.54,22.23 v32.7,22.38 | 34.92,44.84 R2.1 34.92,45.09 v34.92,45.72 | Q1.3 23.29,45.9 v23.32,45.87
  Bottom 0.254: v32.7,22.38 32.22,22.86 32.22,44.28 32.38,44.45 | v23.32,45.87 26.21,45.87 26.98,46.63 30.2,46.63 32.38,44.45 | 32.38,44.45 33.66,45.72 v34.92,45.72
SCL_3V  (via drill 0.3)
  Top 0.254: Q1.2 26.83,48.32 v27.13,48.62
  Bottom 0.254: v27.13,48.62 27.28,48.77 36.32,48.77 36.83,48.26 36.85,48.26 37.11,48.01 37.11,47.86 JP5.3
SDA  (via drill 0.3)
  Top 0.254: 31.59,20.54 D1.27 31.62,20.5 31.62,21.26 31.74,21.38 v31.74,22.38 | Q2.3 27.73,46.17 v27.58,46.02 | R1.1 30.85,44.72 v30.79,44.65
  Bottom 0.254: v31.74,22.38 31.74,43.69 v30.79,44.65 30.63,44.81 30.63,45.57 30.18,46.02 v27.58,46.02
SDA_3V
  Top 0.254: Q2.2 31.41,48.32 31.85,48.77 33.91,48.77 34.67,48.01 34.67,47.75 JP5.2
TXD  (via drill 0.3)
  Top 0.254: R6.1 29.29,16.35 v29.11,16.54 | 31.17,6.6 D2.5 31.24,6.55 31.24,7.54 31.17,7.62 v31.17,7.92 31.7,7.92 32.84,9.07 36.88,9.07 37.64,8.31 37.64,7.7 38.1,7.24 38.1,3.96 36.68,2.54 JP11.1
  Bottom 0.254: v29.11,16.54 29.11,9.63 29.84,8.89 29.84,8.87 30.79,7.92 v31.17,7.92
VBOOT1
  Top 0.254: D3.18 23.17,15.88 23.65,16.35 C20.1 24.34,17.17 24.54,17.37 26.06,17.37 26.21,17.53 26.21,18.68 D6.2
VBUS  (via drill 0.3)
  Top 0.254: X2.VBUS 43.75,15.54 43.89,15.39 43.89,14.69 v43.65,14.45 | v37.64,15.54 37.64,16.19 C11.1
  Top 0.305: v43.65,14.45 v39.36,14.45 | V2.1 44.45,32.38 v45.08,32.38
  Bottom 0.254: v39.36,14.45 38.59,14.45 37.64,15.39 v37.64,15.54
  Bottom 0.305: v43.65,14.45 43.33,14.76 43.33,22.38 45.55,24.61 45.55,31.91 v45.08,32.38
VCC  (via drill 0.3, 0.41, 0.5, 0.6)
  Top 0.406: 31.13,36.2 31.13,37.01 32.22,38.1 34.76,38.1 35.4,38.73 C24.1 | C25.1 C6.+ | C7.+ 30.79,35.35 31.55,34.59 33.68,34.59 36.58,31.7 38.64,31.7 V1.A | v24.38,33.68 24.38,32.64 24.13,32.38 | v23.33,43.81 23.33,42.34 D5.1 | D6.1 23.22,19.84 19.84,19.84 v19.68,19.68
  Top 0.813: D3.9 10.31,8.26 | D4.9 v10.31,32.38 | v19.84,32.38 D4.12 24.13,32.38 27.36,32.38 30.02,35.05 30.49,35.05 30.79,35.35 | 10.31,8.26 10.31,19.68 v10.15,19.84 10.15,22.68 C6.+ | 10.31,8.26 10.31,2.86 v10.63,2.54 | D3.12 23.33,8.26 v23.65,7.94 | C6.+ 12.24,25.06 | 31.13,36.2 C7.+ | C6.+ 9.06,27.94 v8.89,27.94 5.71,27.94 3.01,30.64 F1.P$2
  Bottom 0.406: v23.33,43.81 23.33,34.73 v24.38,33.68 | v19.68,19.68 10.31,19.68 v10.15,19.84
  Bottom 0.813: v19.84,32.38 19.84,31.43 18.89,30.48 12.54,30.48 11.58,31.43 10.31,31.43 | v10.31,32.38 10.31,31.43 | 10.31,31.43 10.31,29.36 v8.89,27.94 | v23.65,7.94 23.65,5.23 20.95,2.54 v10.63,2.54
VCC_VI
  Top 0.406: C4.2 37.3,39.1 37.3,37.47 38.42,36.34 V1.C 39.03,36.2 39.37,36.2 39.88,37.01 V7.3
VCP1
  Top 0.254: D6.3 25.48,20.73 26.52,20.73 27.43,19.81 27.43,15.75 C18.1

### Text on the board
tNames: +5V SDA.SCL.GND.INT | ROLL | GndPitchRoll | Multi 5V GND | + | - | PITCH | TXD RXD 5V GND | AVR / SPI
tStop: M | K | : | ) | by Martinez | FPV-Community
bStop: Brushlessgimbal.de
